| IBIS file stm32u073_083_wlcsp42.ibs
[IBIS ver] 4.2
[File name] stm32u073_083_wlcsp42.ibs
[File Rev] 0.3
[Date] 20-02-2024
[Source] Data Created at STMicroelectronics
[Notes]  File originated from ELDO simulations.
[Disclaimer]  This information is for modeling purpose only and is
   not guaranteed. The information is subject to change without
   notice.
[Copyright] Copyright 2024 STMicroelectronics Inc.
|   Component stm32u073_083_wlcsp42
[Component] stm32u073_083_wlcsp42
[Manufacturer] STMicroelectronics
[Package]
| variable   typ   min   max
R_pkg  0  NA  NA
L_pkg  0  NA  NA
C_pkg  0  NA  NA
[Pin]   signal_name   model_name
A2  VSS  gnd
A4  PA15  io8_ft
A6  PB5  io8_ft
A8  PB7  io8_ft_i2c
A10  PB8  io8_ft_i2c
A12  VSS  gnd
B1  VDDUSB  power
B3  PA13  io8_ft
B5  PB3  io8_ft_i2c
B7  PB6  io8_ft_i2c
B9  VBAT  power
B11  VDD  power
C2  PA12  io8usb_ft_phy
C4  PA9  io8_ft_i2c
C6  PB4  io8_ft_i2c
C8  PF3-BOOT0  io8_ft_v33
C10  PC15-OSC32_OUT  io8_ft
C12  PC14-OSC32_IN  io8_ft_v33
D1  PA11  io8usb_ft_phy
D3  PA8  io8_ft
D5  PA14  io8_ft
D7  PC13  io8_ft_v33
D9  PF1-OSC_OUT  io8_ft
D11  PF0-OSC_IN  io8_ft
E2  PA10  io8_ft_i2c
E4  PA5  io8_ft
E6  PA3  io8_ft
E8  PA1  io8_ft_v33
E10  VSSA_VREFM  nc
E12  PF2-NRST  ioreset_ft_v33
F1  VSS  gnd
F3  PB1  io8_ft
F5  PB0  io8_ft
F7  PA7  io8_ft_i2c
F9  PA0  io8_ft_v33
F11  VDDA_VREFP  nc
G2  VDD  power
G4  PB10  io8_ft_i2c
G6  PB2  io8_ft
G8  PA6  io8_ft_i2c
G10  PA4  io8_ft
G12  PA2  io8_ft_v33
[Package Model]   489-wlcsp-42-240123
[Pin Mapping]   pulldown_ref   pullup_ref   | Comment
A2  gndio  nc
A4  gndio  vddio
A6  gndio  vddio
A8  gndio  vddio
A10  gndio  vddio
A12  gndio  nc
B1  nc  vddusb
B3  gndio  vddio
B5  gndio  vddio
B7  gndio  vddio
B9  nc  vsw
B11  nc  vddio
C2  gndio  vddusb  | Depending on IO usage
| C2  gndio  vddio  | Depending on IO usage
C4  gndio  vddio
C6  gndio  vddio
C8  gndio  vddio
C10  gndio  vddio  | Depending on IO usage
| C10  gndio  vsw  | Depending on IO usage
C12  gndio  vddio  | Depending on IO usage
| C12  gndio  vsw  | Depending on IO usage
D1  gndio  vddusb  | Depending on IO usage
| D1  gndio  vddio  | Depending on IO usage
D3  gndio  vddio
D5  gndio  vddio
D7  gndio  vddio  | Depending on IO usage
| D7  gndio  vsw  | Depending on IO usage
D9  gndio  vddio
D11  gndio  vddio
E2  gndio  vddio
E4  gndio  vddio
E6  gndio  vddio
E8  gndio  vddio
E10  nc  nc
E12  gndio  vddio
F1  gndio  nc
F3  gndio  vddio
F5  gndio  vddio
F7  gndio  vddio
F9  gndio  vddio
F11  nc  nc
G2  nc  vddio
G4  gndio  vddio
G6  gndio  vddio
G8  gndio  vddio
G10  gndio  vddio
G12  gndio  vddio
|[Diff Pin]   inv_pin   vdiff   tdelay_typ   tdelay_min   tdelay_max
|C2   D1   NA   NA   NA   NA
[Model Selector] io8_ft
io8_ft_ls_1v2   "GPIO - 5V tolerant - 1.2V range - Low speed"
io8_ft_ms_1v2   "GPIO - 5V tolerant - 1.2V range - Med speed"
io8_ft_fs_1v2   "GPIO - 5V tolerant - 1.2V range - Fast speed"
io8_ft_hs_1v2   "GPIO - 5V tolerant - 1.2V range - High speed"
io8_ft_ls_1v8   "GPIO - 5V tolerant - 1.8V range - Low speed"
io8_ft_ms_1v8   "GPIO - 5V tolerant - 1.8V range - Med speed"
io8_ft_fs_1v8   "GPIO - 5V tolerant - 1.8V range - Fast speed"
io8_ft_hs_1v8   "GPIO - 5V tolerant - 1.8V range - High speed"
io8_ft_ls_3v3   "GPIO - 5V tolerant - 3.3V range - Low speed"
io8_ft_ms_3v3   "GPIO - 5V tolerant - 3.3V range - Med speed"
io8_ft_fs_3v3   "GPIO - 5V tolerant - 3.3V range - Fast speed"
io8_ft_hs_3v3   "GPIO - 5V tolerant - 3.3V range - High speed"
[Model Selector] io8_ft_i2c
io8_ft_ls_1v2   "GPIO - 5V tolerant - 1.2V range - Low speed"
io8_ft_ms_1v2   "GPIO - 5V tolerant - 1.2V range - Med speed"
io8_ft_fs_1v2   "GPIO - 5V tolerant - 1.2V range - Fast speed"
io8_ft_hs_1v2   "GPIO - 5V tolerant - 1.2V range - High speed"
io8_ft_ls_1v8   "GPIO - 5V tolerant - 1.8V range - Low speed"
io8_ft_ms_1v8   "GPIO - 5V tolerant - 1.8V range - Med speed"
io8_ft_fs_1v8   "GPIO - 5V tolerant - 1.8V range - Fast speed"
io8_ft_hs_1v8   "GPIO - 5V tolerant - 1.8V range - High speed"
io8_ft_ls_3v3   "GPIO - 5V tolerant - 3.3V range - Low speed"
io8_ft_ms_3v3   "GPIO - 5V tolerant - 3.3V range - Med speed"
io8_ft_fs_3v3   "GPIO - 5V tolerant - 3.3V range - Fast speed"
io8_ft_hs_3v3   "GPIO - 5V tolerant - 3.3V range - High speed"
io8_ft_i2c_ls_1v2   "GPIO I2C open-drain - 5V tolerant - 1.2V range - Low speed"
io8_ft_i2c_ms_1v2   "GPIO I2C open-drain - 5V tolerant - 1.2V range - Med speed"
io8_ft_i2c_fs_1v2   "GPIO I2C open-drain - 5V tolerant - 1.2V range - Fast speed"
io8_ft_i2c_hs_1v2   "GPIO I2C open-drain - 5V tolerant - 1.2V range - High speed"
io8_ft_i2c_ls_1v8   "GPIO I2C open-drain - 5V tolerant - 1.8V range - Low speed"
io8_ft_i2c_ms_1v8   "GPIO I2C open-drain - 5V tolerant - 1.8V range - Med speed"
io8_ft_i2c_fs_1v8   "GPIO I2C open-drain - 5V tolerant - 1.8V range - Fast speed"
io8_ft_i2c_hs_1v8   "GPIO I2C open-drain - 5V tolerant - 1.8V range - High speed"
io8_ft_i2c_ls_3v3   "GPIO I2C open-drain - 5V tolerant - 3.3V range - Low speed"
io8_ft_i2c_ms_3v3   "GPIO I2C open-drain - 5V tolerant - 3.3V range - Med speed"
io8_ft_i2c_fs_3v3   "GPIO I2C open-drain - 5V tolerant - 3.3V range - Fast speed"
io8_ft_i2c_hs_3v3   "GPIO I2C open-drain - 5V tolerant - 3.3V range - High speed"
io8_ft_i2c_fmp_3v3   "GPIO I2C open-drain fm+ - 5V tolerant - 3.3V range"
[Model Selector] io8_ft_v33
io8_ft_v33_ls_1v2   "GPIO_V33 - 5V tolerant - 1.2V range - Low speed"
io8_ft_v33_ms_1v2   "GPIO_V33 - 5V tolerant - 1.2V range - Med speed"
io8_ft_v33_fs_1v2   "GPIO_V33 - 5V tolerant - 1.2V range - Fast speed"
io8_ft_v33_hs_1v2   "GPIO_V33 - 5V tolerant - 1.2V range - High speed"
io8_ft_v33_ls_1v8   "GPIO_V33 - 5V tolerant - 1.8V range - Low speed"
io8_ft_v33_ms_1v8   "GPIO_V33 - 5V tolerant - 1.8V range - Med speed"
io8_ft_v33_fs_1v8   "GPIO_V33 - 5V tolerant - 1.8V range - Fast speed"
io8_ft_v33_hs_1v8   "GPIO_V33 - 5V tolerant - 1.8V range - High speed"
io8_ft_v33_ls_3v3   "GPIO_V33 - 5V tolerant - 3.3V range - Low speed"
io8_ft_v33_ms_3v3   "GPIO_V33 - 5V tolerant - 3.3V range - Med speed"
io8_ft_v33_fs_3v3   "GPIO_V33 - 5V tolerant - 3.3V range - Fast speed"
io8_ft_v33_hs_3v3   "GPIO_V33 - 5V tolerant - 3.3V range - High speed"
[Model Selector] io8usb_ft_phy
io8_ft_ls_1v2   "GPIO - 5V tolerant - 1.2V range - Low speed"
io8_ft_ms_1v2   "GPIO - 5V tolerant - 1.2V range - Med speed"
io8_ft_fs_1v2   "GPIO - 5V tolerant - 1.2V range - Fast speed"
io8_ft_hs_1v2   "GPIO - 5V tolerant - 1.2V range - High speed"
io8_ft_ls_1v8   "GPIO - 5V tolerant - 1.8V range - Low speed"
io8_ft_ms_1v8   "GPIO - 5V tolerant - 1.8V range - Med speed"
io8_ft_fs_1v8   "GPIO - 5V tolerant - 1.8V range - Fast speed"
io8_ft_hs_1v8   "GPIO - 5V tolerant - 1.8V range - High speed"
io8_ft_ls_3v3   "GPIO - 5V tolerant - 3.3V range - Low speed"
io8_ft_ms_3v3   "GPIO - 5V tolerant - 3.3V range - Med speed"
io8_ft_fs_3v3   "GPIO - 5V tolerant - 3.3V range - Fast speed"
io8_ft_hs_3v3   "GPIO - 5V tolerant - 3.3V range - High speed"
io8usb_ft_phy_hs_3v3   "USB full speed"
io8usb_ft_phy_ls_3v3   "USB low speed"
[Model Selector] ioreset_ft_v33
ioreset_ft_v33_1v2   "Reset PAD. 5V tolerant. 1.2V range"
ioreset_ft_v33_1v8   "Reset PAD. 5V tolerant. 1.8V range"
ioreset_ft_v33_3v3   "Reset PAD. 5V tolerant. 3.3V range"
[Define Package Model]  489-wlcsp-42-240123
[Manufacturer]  Unknown
[OEM]  Unknown
[Description]  None
[Number Of Pins]  40
[Pin Numbers]
| Pin Num   Terminal Name
F9 | PA0
E8 | PA1
G12 | PA2
E6 | PA3
G10 | PA4
E4 | PA5
G8 | PA6
F7 | PA7
D3 | PA8
C4 | PA9
E2 | PA10
D1 | PA11
C2 | PA12
B3 | PA13
D5 | PA14
A4 | PA15
F5 | PB0
F3 | PB1
G6 | PB2
B5 | PB3
C6 | PB4
A6 | PB5
B7 | PB6
A8 | PB7
A10 | PB8
G4 | PB10
D7 | PC13
C12 | PC14-OSC32_IN
C10 | PC15-OSC32_OUT
D11 | PF0-OSC_IN
D9 | PF1-OSC_OUT
E12 | PF2-NRST
C8 | PF3-BOOT0
B9 | VBAT
B11 | VDD
F11 | VDDA_VREFP
B1 | VDDUSB
A2 | VSS
F1 | VSS
E10 | VSSA_VREFM
|[Merged Pins]  B11
|G2  |  VDD
|[Merged Pins]  A2
|A12  |  VSS
[Model Data]
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[End Model Data]
[End Package Model]
|End [Component]
| Models and submodels in the file (42): io8_ft_fs_1v2 (I/O), io8_ft_fs_1v8 (I/O), io8_ft_fs_3v3 (I/O), io8_ft_hs_1v2 (I/O), io8_ft_hs_1v8 (I/O), io8_ft_hs_3v3 (I/O), io8_ft_i2c_fmp_3v3 (I/O_open_drain), io8_ft_i2c_fs_1v2 (I/O_open_drain), io8_ft_i2c_fs_1v8 (I/O_open_drain), io8_ft_i2c_fs_3v3 (I/O_open_drain), io8_ft_i2c_hs_1v2 (I/O_open_drain), io8_ft_i2c_hs_1v8 (I/O_open_drain), io8_ft_i2c_hs_3v3 (I/O_open_drain), io8_ft_i2c_ls_1v2 (I/O_open_drain), io8_ft_i2c_ls_1v8 (I/O_open_drain), io8_ft_i2c_ls_3v3 (I/O_open_drain), io8_ft_i2c_ms_1v2 (I/O_open_drain), io8_ft_i2c_ms_1v8 (I/O_open_drain), io8_ft_i2c_ms_3v3 (I/O_open_drain), io8_ft_ls_1v2 (I/O), io8_ft_ls_1v8 (I/O), io8_ft_ls_3v3 (I/O), io8_ft_ms_1v2 (I/O), io8_ft_ms_1v8 (I/O), io8_ft_ms_3v3 (I/O), io8_ft_v33_fs_1v2 (I/O), io8_ft_v33_fs_1v8 (I/O), io8_ft_v33_fs_3v3 (I/O), io8_ft_v33_hs_1v2 (I/O), io8_ft_v33_hs_1v8 (I/O), io8_ft_v33_hs_3v3 (I/O), io8_ft_v33_ls_1v2 (I/O), io8_ft_v33_ls_1v8 (I/O), io8_ft_v33_ls_3v3 (I/O), io8_ft_v33_ms_1v2 (I/O), io8_ft_v33_ms_1v8 (I/O), io8_ft_v33_ms_3v3 (I/O), io8usb_ft_phy_hs_3v3 (I/O), io8usb_ft_phy_ls_3v3 (I/O), ioreset_ft_v33_1v2 (I/O_open_drain), ioreset_ft_v33_1v8 (I/O_open_drain), ioreset_ft_v33_3v3 (I/O_open_drain)
